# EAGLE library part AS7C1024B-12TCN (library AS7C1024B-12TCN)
Industrial and commercial temperatures Organization: 131,072 words x 8 bits High speed 10/12/15/20 ns address access time 5/6/7/8 ns output enable access time Low power consumption: ACTIVE 605 mW / max @ 10 ns Low power consumption: STANDBY 55 mW / max CMOS Easy memory expansion with CE1, CE2, OE inputs TTL/LVTTL-compatible, three-state I/O 32-pin JEDEC standard packages Source: Datasheet
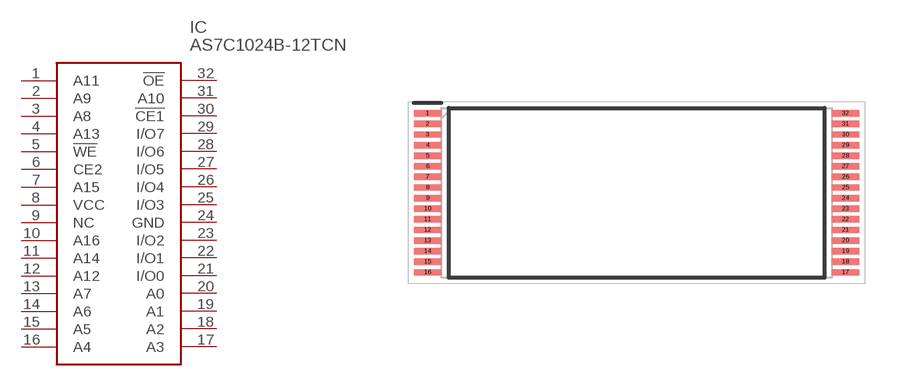
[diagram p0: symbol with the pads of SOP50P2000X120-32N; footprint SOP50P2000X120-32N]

Designator prefix IC

## AS7C1024B-12TCN (Description: Industrial and commercial temperatures Organization: 131,072 words x 8 bits High speed 10/12/15/20 ns address access time 5/6/7/8 ns output enable access time Low power consumption: ACTIVE 605 mW / max @ 10 ns Low power consumption: STANDBY 55 mW / max CMOS Easy memory expansion with CE1, CE2, OE inputs TTL/LVTTL-compatible, three-state I/O 32-pin JEDEC standard packages; Height: 1.2mm; Manufacturer_Name: Alliance Memory; Manufacturer_Part_Number: AS7C1024B-12TCN; Mouser_Part_Number: 913-AS7C1024B-12TCN; Mouser_Price-Stock: https://www.mouser.co.uk/ProductDetail/Alliance-Memory/AS7C1024B-12TCN?qs=E5c5%252Bmu3i39p9b7hUnTiBw%3D%3D)  [SOP50P2000X120-32N]
1  A11
2  A9
3  A8
4  A13
5  !WE
6  CE2
7  A15
8  VCC
9  NC  nc
10  A16
11  A14
12  A12
13  A7
14  A6
15  A5
16  A4
17  A3
18  A2
19  A1
20  A0
21  I/O0
22  I/O1
23  I/O2
24  GND
25  I/O3
26  I/O4
27  I/O5
28  I/O6
29  I/O7
30  !CE1
31  A10
32  !OE

## Footprint SOP50P2000X120-32N (pad centres in mm)
32-pin TSOP 8&times;20 mm
smd 1.3 x 0.3: 1 -9.85,3.75; 2 -9.85,3.25; 3 -9.85,2.75; 4 -9.85,2.25; 5 -9.85,1.75; 6 -9.85,1.25; 7 -9.85,0.75; 8 -9.85,0.25; 9 -9.85,-0.25; 10 -9.85,-0.75; 11 -9.85,-1.25; 12 -9.85,-1.75; 13 -9.85,-2.25; 14 -9.85,-2.75; 15 -9.85,-3.25; 16 -9.85,-3.75; 17 9.85,-3.75; 18 9.85,-3.25; 19 9.85,-2.75; 20 9.85,-2.25; 21 9.85,-1.75; 22 9.85,-1.25; 23 9.85,-0.75; 24 9.85,-0.25; 25 9.85,0.25; 26 9.85,0.75; 27 9.85,1.25; 28 9.85,1.75; 29 9.85,2.25; 30 9.85,2.75; 31 9.85,3.25; 32 9.85,3.75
